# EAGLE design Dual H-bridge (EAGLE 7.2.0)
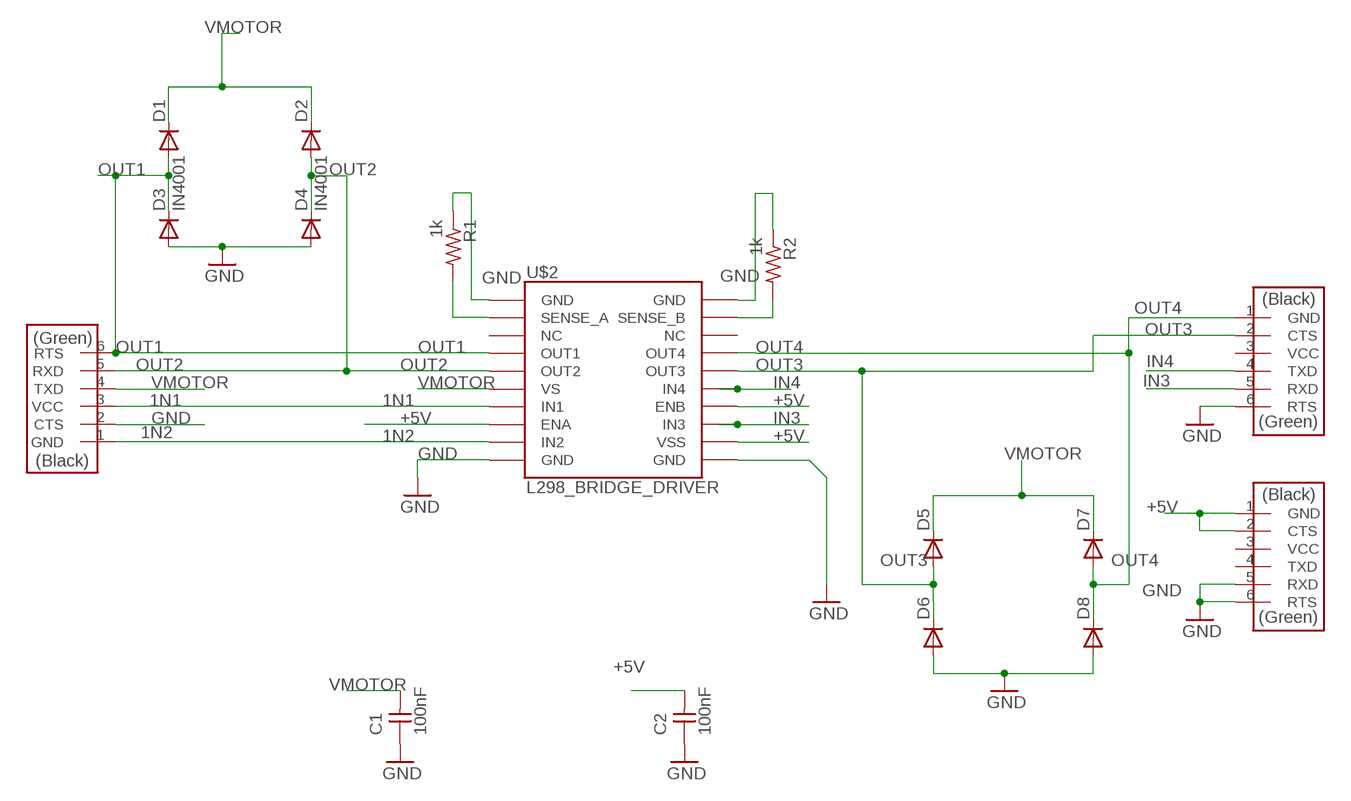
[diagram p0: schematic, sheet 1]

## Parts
C1  100nF  CAP-UNPOLARIZEDFAB  [C1206FAB]
C2  100nF  CAP-UNPOLARIZEDFAB  [C1206FAB]
D1  DIODESMA  [SMA-DIODE]
D2  DIODESMA  [SMA-DIODE]
D3  IN4001  DIODESMA  [SMA-DIODE]
D4  IN4001  DIODESMA  [SMA-DIODE]
D5  DIODESMA  [SMA-DIODE]
D6  DIODESMA  [SMA-DIODE]
D7  DIODESMA  [SMA-DIODE]
D8  DIODESMA  [SMA-DIODE]
R1  1k  RES-US1206FAB  [R1206FAB]
R2  1k  RES-US1206FAB  [R1206FAB]
U$1  FTDI-SMD-HEADER  [1X06SMD]
U$2  L298_BRIDGE_DRIVER  [POWERSO20]
U$3  FTDI-SMD-HEADER  [1X06SMD]
U$6  FTDI-SMD-HEADER  [1X06SMD]

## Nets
1N1: U$1.3(VCC) U$2.P$7(IN1)
1N2: U$1.1(GND) U$2.P$9(IN2)
+5V: C2.2 U$2.P$8(ENA) U$2.P$12(VSS) U$2.P$14(ENB) U$3.1(GND) U$3.2(CTS)
GND: C1.1 C2.1 D3.A D4.A D6.A D8.A R1.1 R2.1 U$1.2(CTS) U$2.P$1(GND) U$2.P$10(GND) U$2.P$11(GND) U$2.P$20(GND) U$3.5(RXD) U$3.6(RTS) U$6.6(RTS)
IN3: U$2.P$13(IN3) U$6.5(RXD)
IN4: U$2.P$15(IN4) U$6.4(TXD)
N$2: R1.2 U$2.P$2(SENSE_A)
N$3: R2.2 U$2.P$19(SENSE_B)
OUT1: D1.A D3.C U$1.6(RTS) U$2.P$4(OUT1)
OUT2: D2.A D4.C U$1.5(RXD) U$2.P$5(OUT2)
OUT3: D5.A D6.C U$2.P$16(OUT3) U$6.2(CTS)
OUT4: D7.A D8.C U$2.P$17(OUT4) U$6.1(GND)
VMOTOR: C1.2 D1.C D2.C D5.C D7.C U$1.4(TXD) U$2.P$6(VS)
Unconnected: U$2.P$3(NC) U$2.P$18(NC) U$3.3(VCC) U$3.4(TXD) U$6.3(VCC)

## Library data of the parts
C1 C2 = fab-sp:CAP-UNPOLARIZED
D1-D8 = 01_SparkFun:DIODE: Diode
R1 R2 = fab-sp:RES-US: Resistor (US Symbol)
U$1 U$3 U$6 = fab-sp:FTDI-SMD-HEADER
U$2 = 01_SparkFun:L298_BRIDGE_DRIVER

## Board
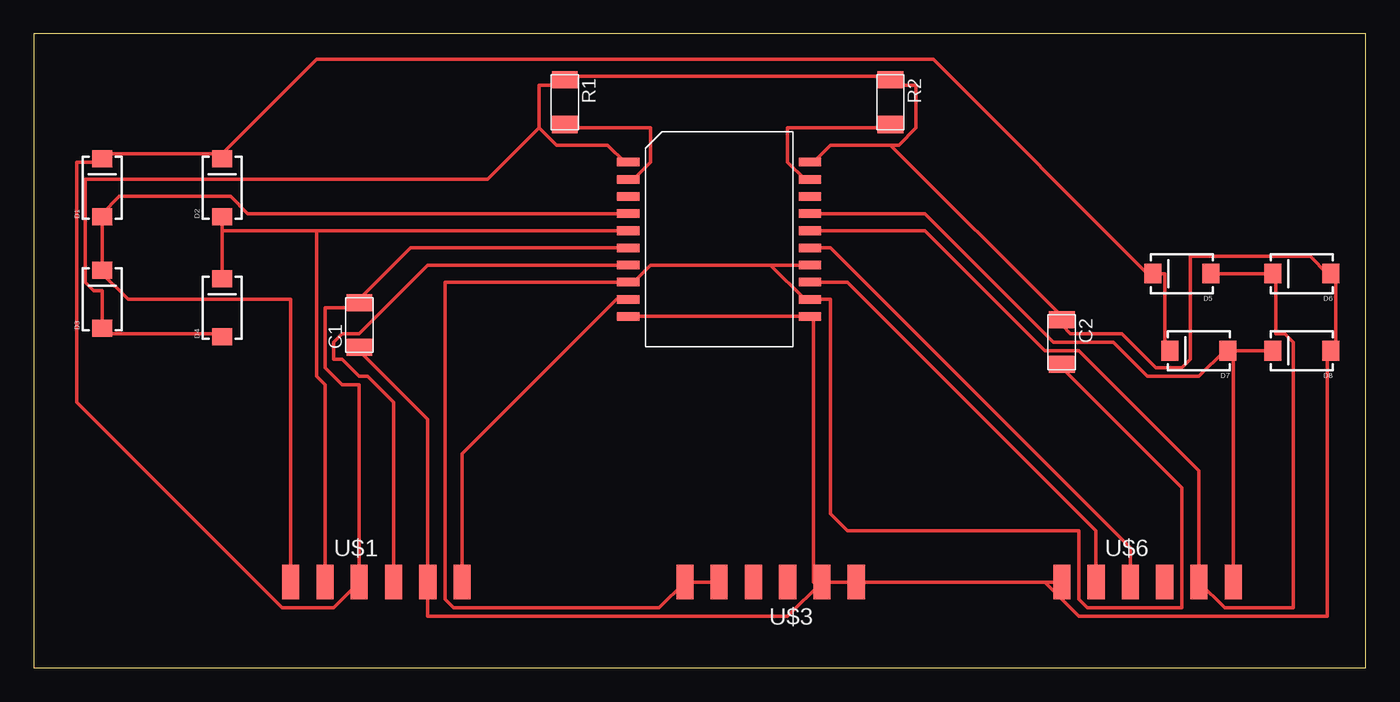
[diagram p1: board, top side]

Size 98.73 x 46.98 mm. Coordinates in mm from the lower left corner, seen from the top.
Outline: 0,0 98.73,0 98.73,46.98 0,46.98 0,0
Copper layers (1*16): Top 0.035mm / dielectric 1.5mm / Bottom 0.035mm
Design rules "default": minimum track width 10mil, minimum drill 24mil, track to track 8mil, track to pad 8mil, pad to pad 8mil, via to via 8mil, smd to smd 8mil, copper to edge 40mil, drill to drill 8mil, minimum pad ring 10mil, minimum via ring 8mil, stop-mask expansion 4mil, vias tented up to drill 0mil, thermal gap 10mil

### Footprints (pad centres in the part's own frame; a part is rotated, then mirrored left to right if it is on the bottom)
C1206FAB = smd 1.27 x 1.905: 1 -1.651,0; 2 1.651,0
SMA-DIODE = smd 1.27 x 1.47: A -2.15,0; C 2.15,0
R1206FAB = smd 1.27 x 1.905: 1 -1.651,0; 2 1.651,0
1X06SMD = smd 2.54 x 1.27: 1 0,6.35; 2 0,3.81; 3 0,1.27; 4 0,-1.27; 5 0,-3.81; 6 0,-6.35
POWERSO20 = smd 1.651 x 0.635: P$1 -6.731,5.715; P$2 -6.731,4.445; P$3 -6.731,3.175; P$4 -6.731,1.905; P$5 -6.731,0.635; P$6 -6.731,-0.635; P$7 -6.731,-1.905; P$8 -6.731,-3.175; P$9 -6.731,-4.445; P$10 -6.731,-5.715; P$11 6.731,-5.715; P$12 6.731,-4.445; P$13 6.731,-3.175; P$14 6.731,-1.905; P$15 6.731,-0.635; P$16 6.731,0.635; P$17 6.731,1.905; P$18 6.731,3.175; P$19 6.731,4.445; P$20 6.731,5.715

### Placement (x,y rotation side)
C1  24.13,25.4 90 top
C2  76.2,24.13 270 top
D1  5.08,35.56 90 top
D2  13.97,35.56 90 top
D3  5.08,27.3 90 top
D4  13.97,26.67 90 top
D5  85.09,29.21 180 top
D6  93.98,29.21 180 top
D7  86.36,23.49 180 top
D8  93.98,23.49 180 top
R1  39.37,41.91 270 top
R2  63.5,41.91 270 top
U$1  25.4,6.35 270 top
U$2  50.8,31.75 0 top
U$3  54.61,6.35 90 top
U$6  82.55,6.35 270 top

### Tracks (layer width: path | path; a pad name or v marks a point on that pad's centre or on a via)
1N1
  Top 0.254: U$2.P$7 29.21,29.84 24.13,24.77 22.86,24.77 22.23,24.13 22.23,22.86 22.86,22.86 24.13,21.59 24.77,21.59 26.67,19.69 U$1.3
1N2
  Top 0.254: U$2.P$9 43.18,27.3 31.75,15.88 U$1.1
+5V
  Top 0.254: U$3.2 U$3.1 46.36,4.45 31.12,4.45 30.48,5.08 30.48,28.57 U$2.P$8 44.45,28.57 45.72,29.84 54.61,29.84 | U$2.P$14 54.61,29.84 | 54.61,29.84 57.15,27.3 U$2.P$12 59.05,27.3 59.05,11.43 60.33,10.16 77.47,10.16 77.47,5.08 78.1,4.45 85.09,4.45 85.09,13.33 76.2,22.23 C2.2
GND
  Top 0.254: 63.5,38.73 64.13,38.73 65.4,40 65.4,43.18 63.5,43.18 R2.1 63.5,43.81 39.37,43.81 R1.1 39.37,43.18 37.47,43.18 37.47,40 | 63.5,38.73 59.05,38.73 57.79,37.46 U$2.P$20 | 63.5,38.73 76.2,26.03 C2.1 76.2,25.4 76.83,24.77 80.64,24.77 83.18,22.23 85.09,22.23 85.72,22.86 85.72,30.48 94.61,30.48 95.88,29.21 D6.A 96.52,29.21 96.52,23.49 D8.A 95.88,23.49 95.88,3.81 77.47,3.81 74.93,6.35 | D4.A 13.97,24.77 5.08,24.77 D3.A 5.08,27.94 4.45,27.94 3.81,28.57 3.81,36.2 33.66,36.2 37.47,40 | 37.47,40 38.73,38.73 42.55,38.73 43.81,37.46 U$2.P$1 | C1.1 24.13,23.49 29.21,18.41 U$1.2 29.21,3.81 55.88,3.81 U$3.5 | U$2.P$10 U$2.P$11 57.79,26.03 57.79,6.35 U$3.5 | U$3.5 U$3.6 74.93,6.35 | 74.93,6.35 U$6.6
IN3
  Top 0.254: U$2.P$13 60.33,28.57 78.74,10.16 U$6.5
IN4
  Top 0.254: U$2.P$15 59.05,31.12 81.28,8.89 U$6.4
N$2
  Top 0.254: U$2.P$2 44.45,36.2 45.72,37.46 45.72,40 39.37,40 R1.2
N$3
  Top 0.254: U$2.P$19 57.15,36.2 55.88,37.46 55.88,40 63.5,40 R2.2
OUT1
  Top 0.254: U$2.P$4 15.88,33.66 14.61,34.92 6.35,34.92 5.08,33.66 D1.A D3.C 5.08,29.21 6.99,27.3 19.05,27.3 U$1.6
OUT2
  Top 0.254: D2.A 13.97,32.38 | 13.97,32.38 D4.C | 13.97,32.38 20.96,32.38 | 20.96,32.38 U$2.P$5 | U$1.5 21.59,20.95 20.96,21.59 20.96,32.38
OUT3
  Top 0.254: D5.A D6.C 92.07,29.21 92.07,24.77 92.71,24.77 93.34,24.13 93.34,4.45 88.27,4.45 U$6.2 86.36,14.6 77.47,23.49 74.93,23.49 66.04,32.38 U$2.P$16
OUT4
  Top 0.254: D8.C 88.9,23.49 | U$2.P$17 66.04,33.66 75.56,24.13 80.01,24.13 82.55,21.59 86.36,21.59 88.27,23.49 D7.A 88.9,23.49 | 88.9,23.49 U$6.1
VMOTOR
  Top 0.254: U$2.P$6 27.94,31.12 24.13,27.3 C1.2 24.13,26.67 21.59,26.67 21.59,22.23 22.86,20.95 24.13,20.95 U$1.4 22.23,4.45 18.41,4.45 3.17,19.69 3.17,37.46 5.08,37.46 D1.C 5.08,38.1 13.97,38.1 | D7.C 83.82,23.49 83.82,29.21 D5.C 82.55,29.21 66.67,45.09 20.96,45.09 13.97,38.1 | 13.97,38.1 D2.C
